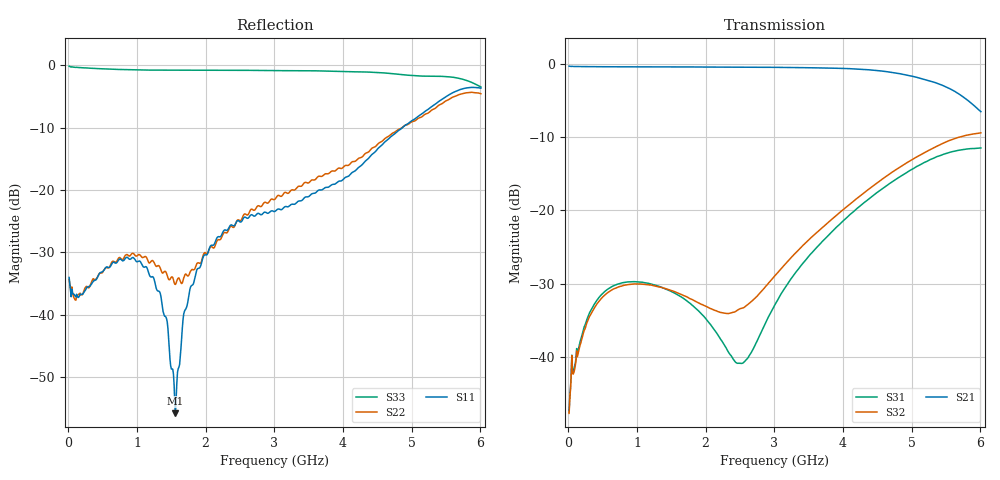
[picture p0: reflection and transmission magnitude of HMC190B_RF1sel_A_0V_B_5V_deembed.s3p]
! Device:	HMC190B
! Description:	GaAs MMIC SPDT Reflective Switch
! Package:	8-lead mini small outline package
! Frequency:	DC -  3 GHz
! Ports:
! RFC = Port 1
! RF1 = Port 2
! RF2 = Port 3
! State: RF1 Selected
! Control Voltages:
! A  = 0 V
! B  = 5 V
! Data:	Data was collected using a calibrated network analyzer with AFR software.
!	Fixtures were calculated using AFR and fixturing was applied to collect
!	this Deembedded  S Parameter data of HMC190B.
! Note:	Analog Devices supplies this data as a sample of measured data at the package pin
!	for this product.  Your particular data for this product may vary.
!	Data was taken at 25 degrees C.
!	Analog Devices reserves the right to change this data at anytime.
# Hz S  dB  R 50
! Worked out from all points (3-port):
!   601 points, 10 MHz to 6.01 GHz, reference 50 ohm
!   strongest paths, dB at 10 MHz, 1.51 GHz, 3.01 GHz, 4.51 GHz, 6.01 GHz:
!     S21: -0.3, -0.4, -0.4, -0.9, -6.5
!     S32: -47.7, -31.0, -28.9, -16.2, -9.4
!     S31: -47.5, -31.1, -32.9, -17.5, -11.5
!   lowest |S11| = -55.8 dB at 1.56 GHz (marker M1), VSWR 1.00, Z = 50.1 - j0.143 ohm
!   |S11| at or under -10 dB: start of sweep to 4.867 GHz
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1e7  -34.01 -5.2  -0.29 -0.5  -47.27 14.1
     -0.28 -0.5  -34.33 -8.4  -47.54 16.7
     -47.48 16.1  -47.71 16.2  -0.14 -2.7
4.8e8  -33.17 45.8  -0.36 -9.8  -31.51 30.2
       -0.36 -9.8  -33.31 39.0  -32.02 38.6
       -31.51 30.2  -32.02 38.5  -0.56 -88.0
1.23e9  -33.89 45.8  -0.38 -25.0  -30.09 -11.6
        -0.38 -25.0  -31.33 22.4  -30.24 14.6
        -30.11 -11.6  -30.24 14.7  -0.78 -157.6
1.56e9  -55.80 -61.7  -0.38 -31.8  -31.37 -26.8
        -0.38 -31.8  -35.13 -27.8  -31.14 11.7
        -31.36 -26.7  -31.14 11.7  -0.79 -174.9
1.69e9  -39.46 -134.7  -0.39 -34.5  -32.10 -33.2
        -0.39 -34.5  -33.79 -56.8  -31.66 12.2
        -32.09 -33.2  -31.66 12.2  -0.79 179.4
1.97e9  -30.58 -142.5  -0.40 -40.4  -34.42 -48.7
        -0.40 -40.4  -30.26 -99.2  -32.95 18.1
        -34.44 -49.1  -32.95 18.1  -0.79 168.4
2.49e9  -25.02 -153.4  -0.42 -51.6  -40.91 -122.2
        -0.42 -51.6  -24.86 -123.1  -33.44 50.5
        -40.87 -122.3  -33.45 50.3  -0.79 151.3
3.01e9  -23.41 -162.8  -0.44 -63.3  -32.84 148.8
        -0.44 -63.3  -21.46 -139.1  -28.90 76.6
        -32.85 148.7  -28.89 76.5  -0.86 135.9
4.47e9  -13.87 157.6  -0.86 -102.2  -17.73 85.0
        -0.85 -102.1  -13.05 171.6  -16.43 61.9
        -17.74 85.1  -16.42 61.9  -1.14 95.7
6.01e9  -3.67 113.9  -6.49 -147.9  -11.45 15.8
        -6.50 -147.9  -4.56 116.2  -9.39 9.2
        -11.45 15.8  -9.39 9.2  -3.47 66.8
